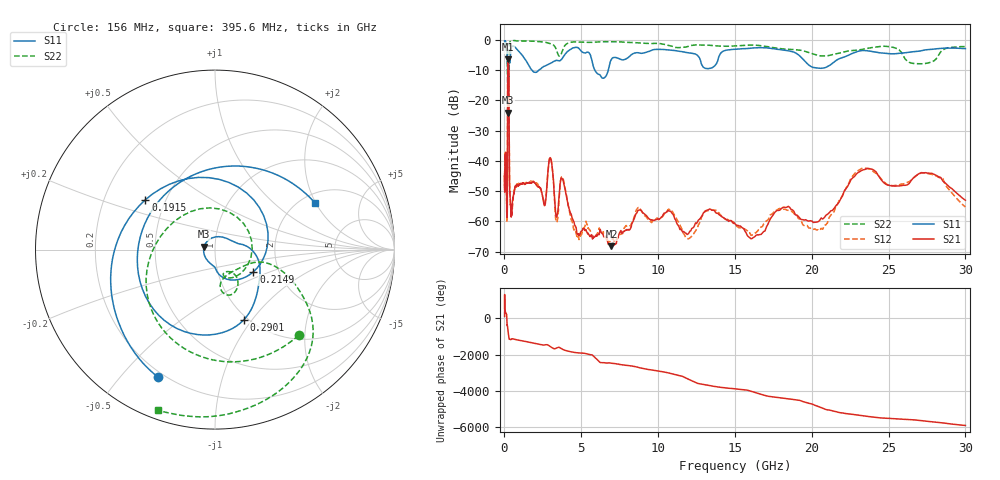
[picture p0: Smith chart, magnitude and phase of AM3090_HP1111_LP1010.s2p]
! Date/Time: Thu, Feb 28, 2019 2:10 PM
! Network Analyzer: Agilent Technologies E8364B Rev: A.07.50.67
! Sweep from 0.010 to 30.000 GHz, 1601 Points, Sweep Type: LOG
! Power Supply: 5.023 V, 0.002 A
# Hz S DB R 50
!freq MagS11 AngS11 MagS21 AngS21 MagS12 AngS12 MagS22 AngS22
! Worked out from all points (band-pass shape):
!   1601 points, 10 MHz to 30 GHz, reference 50 ohm
!   highest |S21| = -6.32 dB at 246 MHz (marker M1); lowest = -68.2 dB at 6.959 GHz (marker M2)
!   |S21| within 3 dB of the highest: 216.9 MHz to 280.8 MHz (63.94 MHz wide, 25.7 % of centre)
!   lowest |S11| = -24.1 dB at 237.5 MHz (marker M3), VSWR 1.13, Z = 44.3 + j1.5 ohm
!   |S11| at or under -10 dB: 206.9 MHz to 272.9 MHz (66.01 MHz wide, 27.5 % of centre); 1.795 GHz to 2.229 GHz (434.4 MHz wide, 21.6 % of centre); 5.885 GHz to 6.755 GHz (870 MHz wide, 13.8 % of centre)
!   |S22| runs from -17.2 to -0.2 dB; largest |S21 - S12| = 0.012
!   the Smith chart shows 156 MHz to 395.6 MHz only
!   S11 on the Smith chart (normalised r, x): 156 MHz: 0.18, -0.64; 191.5 MHz: 0.39, +0.28; 214.9 MHz: 1.48, -0.39; 290.1 MHz: 0.96, -0.91; 395.6 MHz: 2.39, +1.98
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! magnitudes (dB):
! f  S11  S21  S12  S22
! 10 MHz  -0.3  -48.7  -45.0  -0.7
! 38.04 MHz  -0.3  -41.1  -40.5  -1.2
! 105.6 MHz  -1.0  -39.6  -40.4  -3.3
! 144.7 MHz  -1.7  -57.4  -56.9  -3.5
! 156 MHz  -2.2  -56.7  -59.2  -3.5
! 191.5 MHz  -6.4  -45.8  -43.8  -10.6
! 214.9 MHz  -12.1  -10.2  -10.2  -16.4
! 237.5 MHz  -24.1  -6.5  -6.4  -12.7
! 246 MHz  -21.8  -6.3  -6.3  -11.6
! 290.1 MHz  -7.5  -13.4  -13.4  -9.2
! 328.8 MHz  -7.4  -46.8  -46.2  -1.2
! 395.6 MHz  -4.2  -54.7  -54.3  -0.4
! 550.5 MHz  -2.0  -52.2  -53.8  -0.3
! 2.084 GHz  -10.7  -48.0  -47.4  -0.5
! 2.987 GHz  -7.7  -38.9  -38.8  -1.2
! 3.385 GHz  -6.7  -58.6  -60.3  -3.3
! 3.779 GHz  -6.0  -45.9  -45.3  -3.5
! 6.959 GHz  -6.4  -68.2  -65.8  -0.6
! 7.926 GHz  -6.2  -62.7  -61.3  -0.8
! 20.2 GHz  -9.2  -60.3  -62.5  -4.8
! 23.48 GHz  -3.5  -42.8  -42.4  -2.9
! 30 GHz  -2.9  -53.0  -55.2  -2.2
